(* Logix 5000 AddOnInstructionDefinition export Banner_QS18EAF_PD_v4; software revision 33.00 *)

TYPE Banner_QS18EAF_PDI_v4 :   // Process Data for a QS18EAF. This will include event information.
STRUCT
   Output_State : SINT;   // 0 = Inactive, 1 = Active
   Marginal_Signal : SINT;   // 0 = Normal, 1 = Marginal
END_STRUCT
END_TYPE

ADD_ON_INSTRUCTION Banner_QS18EAF_PD_v4   (* revision 4.0, vendor Banner Engineering *)
// Take raw process data and convert it to usable values.
VAR_INPUT
   SINT0 : SINT; {required}
   SINT1 : SINT; {required}
END_VAR
VAR_IN_OUT
   Process_Data : Banner_QS18EAF_PDI_v4; {required}
END_VAR
VAR_INPUT
   Byte_Swap : BOOL; {required}
END_VAR

ROUTINE Logic   (* ladder *)
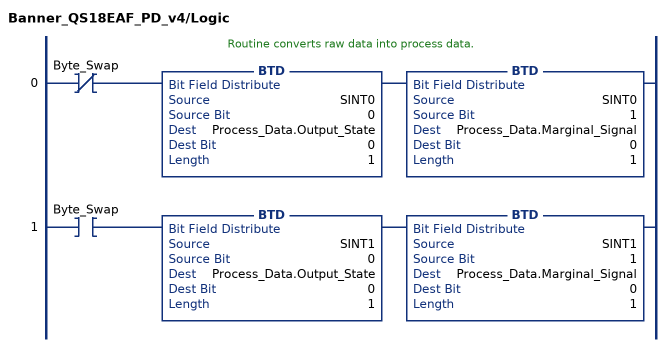
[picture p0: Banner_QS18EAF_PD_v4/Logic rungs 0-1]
   // Routine converts raw data into process data.
   0: XIO(Byte_Swap)BTD(SINT0,0,Process_Data.Output_State,0,1)BTD(SINT0,1,Process_Data.Marginal_Signal,0,1);
   1: XIC(Byte_Swap)BTD(SINT1,0,Process_Data.Output_State,0,1)BTD(SINT1,1,Process_Data.Marginal_Signal,0,1);
END_ROUTINE
END_ADD_ON_INSTRUCTION
